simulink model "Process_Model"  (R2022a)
settings: Solver=ode45  StartTime=0.0  StopTime=300  RelTol=1e-3  EnableMultiTasking=on
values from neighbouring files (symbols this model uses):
  g = 9.81    [init_model.m]
  Ts = 0.05    [init_model.m]
  v = 2    [init_model.m]

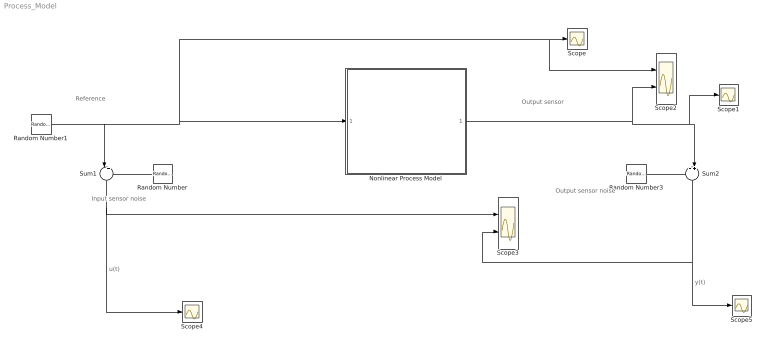
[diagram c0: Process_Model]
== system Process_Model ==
  note: Input sensor noise
  note: Reference
  note: u(t)
  note: Output sensor
  note: y(t)
  note: Output sensor noise
  Nonlinear Process Model : Subsystem
  Random Number : RandomNumber  Variance=0.0001  Seed=1  SampleTime=Ts
  Random Number1 : RandomNumber  Variance=0.1  SampleTime=10
  Random Number3 : RandomNumber  Variance=0.00001  Seed=3  SampleTime=Ts
  Scope{,1,4..5} (4 alike) : Scope
  Scope2 : Scope  NumInputPorts=2
  Scope3 : Scope  NumInputPorts=2
  Sum1 : Sum  Inputs=|++  SaturateOnIntegerOverflow=on
  Sum2 : Sum  Inputs=++|  SaturateOnIntegerOverflow=on
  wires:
  Random Number1/1 -> Sum1/1, Scope2/1, Scope/1, Nonlinear Process Model/1(Force u*(t))
  Sum1/1 -> Scope4/1, Scope3/1
  Nonlinear Process Model/1(Angle y*(t)) -> Scope1/1, Sum2/2, Scope2/2
  Random Number/1 -> Sum1/2
  Random Number3/1 -> Sum2/1
  Sum2/1 -> Scope5/1, Scope3/2

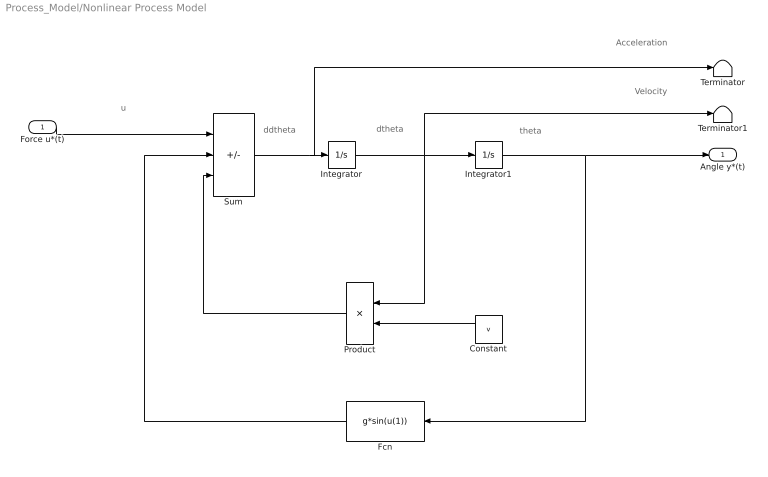
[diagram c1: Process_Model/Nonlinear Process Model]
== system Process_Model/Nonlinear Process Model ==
  note: Velocity
  note: Acceleration
  note: ddtheta
  note: dtheta
  note: theta
  note: u
  Force u*(t) : Inport
  Constant : Constant  Value=v
  Fcn : Fcn  Expr=g*sin(u(1))
  Integrator : Integrator
  Integrator1 : Integrator  InitialCondition=(pi/180)*90
  Product : Product
  Sum : Sum  Inputs=+--  SaturateOnIntegerOverflow=on
  Terminator : Terminator
  Terminator1 : Terminator
  Angle y*(t) : Outport
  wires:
  Sum/1 -> Terminator/1, Integrator/1
  Integrator/1 -> Terminator1/1, Product/1, Integrator1/1
  Integrator1/1 -> Angle y*(t)/1, Fcn/1
  Fcn/1 -> Sum/2
  Product/1 -> Sum/3
  Force u*(t)/1 -> Sum/1
  Constant/1 -> Product/2
